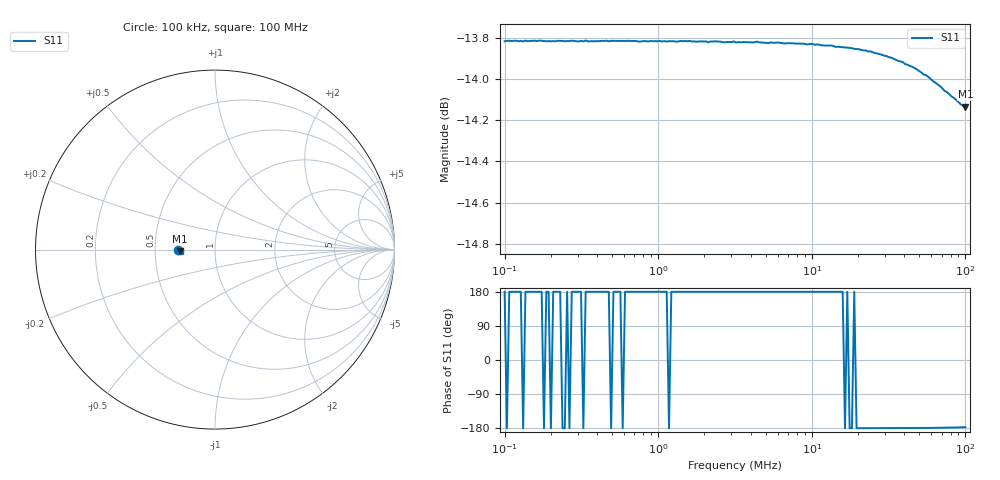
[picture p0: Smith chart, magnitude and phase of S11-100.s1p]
! ListType=Log
!!100 Ohm Shunt
# MHz S RI R 50
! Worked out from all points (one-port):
!   200 points, 100 kHz to 100 MHz, reference 50 ohm
!   lowest |S11| = -14.1 dB at 100 MHz (marker M1), VSWR 1.49, Z = 33.6 - j0.647 ohm
!   |S11| at or under -10 dB: start of sweep to end of sweep
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0.1  -0.2038 3.77e-05
0.2381686  -0.2038 -8.7e-06
0.5672426  -0.2038 4.53e-05
1.350993  -0.2038 6.33e-05
2.049075  -0.2038 8.08e-05
2.121452  -0.2037 0.000131
2.354286  -0.2038 6.61e-05
2.70496  -0.2037 0.000105
3.107866  -0.2038 8.51e-05
3.217642  -0.2037 0.000169
4.397604  -0.2038 0.000159
5.231099  -0.2036 0.000129
5.415871  -0.2037 0.000173
7.663411  -0.2036 0.000118
13.35452  -0.2033 8.15e-05
14.31459  -0.2032 7.33e-05
18.25183  -0.203 -1.57e-05
24.09404  -0.2026 -0.000178
30.72113  -0.2021 -0.000443
39.17101  -0.2014 -0.00098
40.55461  -0.2012 -0.00105
43.47013  -0.201 -0.00126
55.42665  -0.1999 -0.00231
70.67181  -0.1985 -0.0042
73.16807  -0.1982 -0.00457
84.06653  -0.1973 -0.00622
93.29304  -0.1966 -0.00789
100  -0.1962 -0.00926
